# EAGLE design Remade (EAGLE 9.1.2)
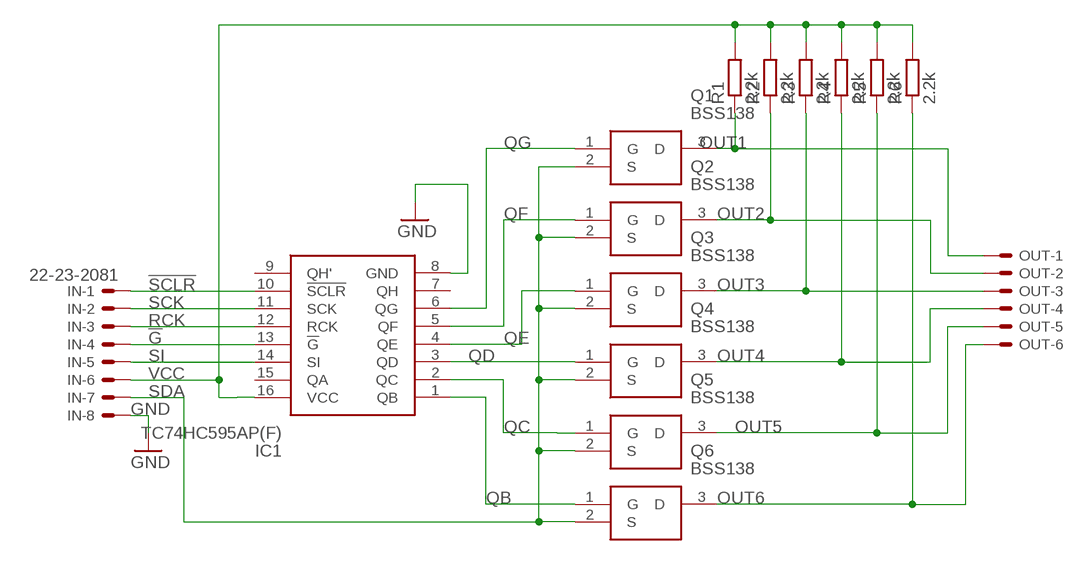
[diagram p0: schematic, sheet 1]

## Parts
IC1  TC74HC595AP(F)  [DIP762W60P254L1925H445Q16N]
IN  22-23-2081  [22-23-2081]
OUT  22-23-2061  [22-23-2061]
Q1  BSS138  [SOT95P240X120-3N]
Q2  BSS138  [SOT95P240X120-3N]
Q3  BSS138  [SOT95P240X120-3N]
Q4  BSS138  [SOT95P240X120-3N]
Q5  BSS138  [SOT95P240X120-3N]
Q6  BSS138  [SOT95P240X120-3N]
R1  2.2k  R-EU_0207/15  [0207/15]
R2  2.2k  R-EU_0207/15  [0207/15]
R3  2.2k  R-EU_0207/15  [0207/15]
R4  2.2k  R-EU_0207/15  [0207/15]
R5  2.2k  R-EU_0207/15  [0207/15]
R6  2.2k  R-EU_0207/15  [0207/15]

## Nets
!G: IC1.13(!G) IN.4
!SCLR: IC1.10(!SCLR) IN.1
GND: IC1.8(GND) IN.8
OUT1: OUT.1 Q1.3(D) R1.1
OUT2: OUT.2 Q2.3(D) R2.1
OUT3: OUT.3 Q3.3(D) R3.1
OUT4: OUT.4 Q4.3(D) R4.1
OUT5: OUT.5 Q5.3(D) R5.1
OUT6: OUT.6 Q6.3(D) R6.1
QB: IC1.1(QB) Q6.1(G)
QC: IC1.2(QC) Q5.1(G)
QD: IC1.3(QD) Q4.1(G)
QE: IC1.4(QE) Q3.1(G)
QF: IC1.5(QF) Q2.1(G)
QG: IC1.6(QG) Q1.1(G)
RCK: IC1.12(RCK) IN.3
SCK: IC1.11(SCK) IN.2
SDA: IN.7 Q1.2(S) Q2.2(S) Q3.2(S) Q4.2(S) Q5.2(S) Q6.2(S)
SI: IC1.14(SI) IN.5
VCC: IC1.16(VCC) IN.6 R1.2 R2.2 R3.2 R4.2 R5.2 R6.2
Unconnected: IC1.7(QH) IC1.9(QH') IC1.15(QA)

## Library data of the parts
IC1 = TC74HC595AP(F):TC74HC595AP(F): IC,CMOS logic,DIP16,SHIFT REGISTERS Source: Datasheet; DESCRIPTION: IC,CMOS logic,DIP16,SHIFT REGISTERS; HEIGHT: 4.45mm; MANUFACTURER_NAME: Toshiba; MANUFACTURER_PART_NUMBER: TC74HC595AP(F); MOUSER_PART_NUMBER: N/A; MOUSER_PRICE-STOCK: https://www.mouser.com/Search/Refine.aspx?Keyword=N%2FA; RS_PART_NUMBER: 5400095P; RS_PRICE-STOCK: http://au.rs-online.com/web/p/products/5400095P
IN = con-molex:22-23-2081: .100" (2.54mm) Center Header - 8 Pin; MF: MOLEX; MPN: 22-23-2081; OC_FARNELL: 1756826; OC_NEWARK: 01C7592
OUT = con-molex:22-23-2061: .100" (2.54mm) Center Header - 6 Pin; MF: MOLEX; MPN: 22-23-2061; OC_FARNELL: 1462922; OC_NEWARK: 27C1933
Q1-Q6 = BSS138:BSS138: N-channel MOSFET,BSS138 0.2A 50V Source: Datasheet; DESCRIPTION: N-channel MOSFET,BSS138 0.2A 50V; HEIGHT: 1.2mm; MANUFACTURER_NAME: ON Semiconductor; MANUFACTURER_PART_NUMBER: BSS138; MOUSER_PART_NUMBER: 512-BSS138; RS_PART_NUMBER: 1241694; RS_PRICE-STOCK: http://uk.rs-online.com/web/p/products/1241694
R1-R6 = rcl:R-EU_: RESISTOR, European symbol; SPICEPREFIX: R

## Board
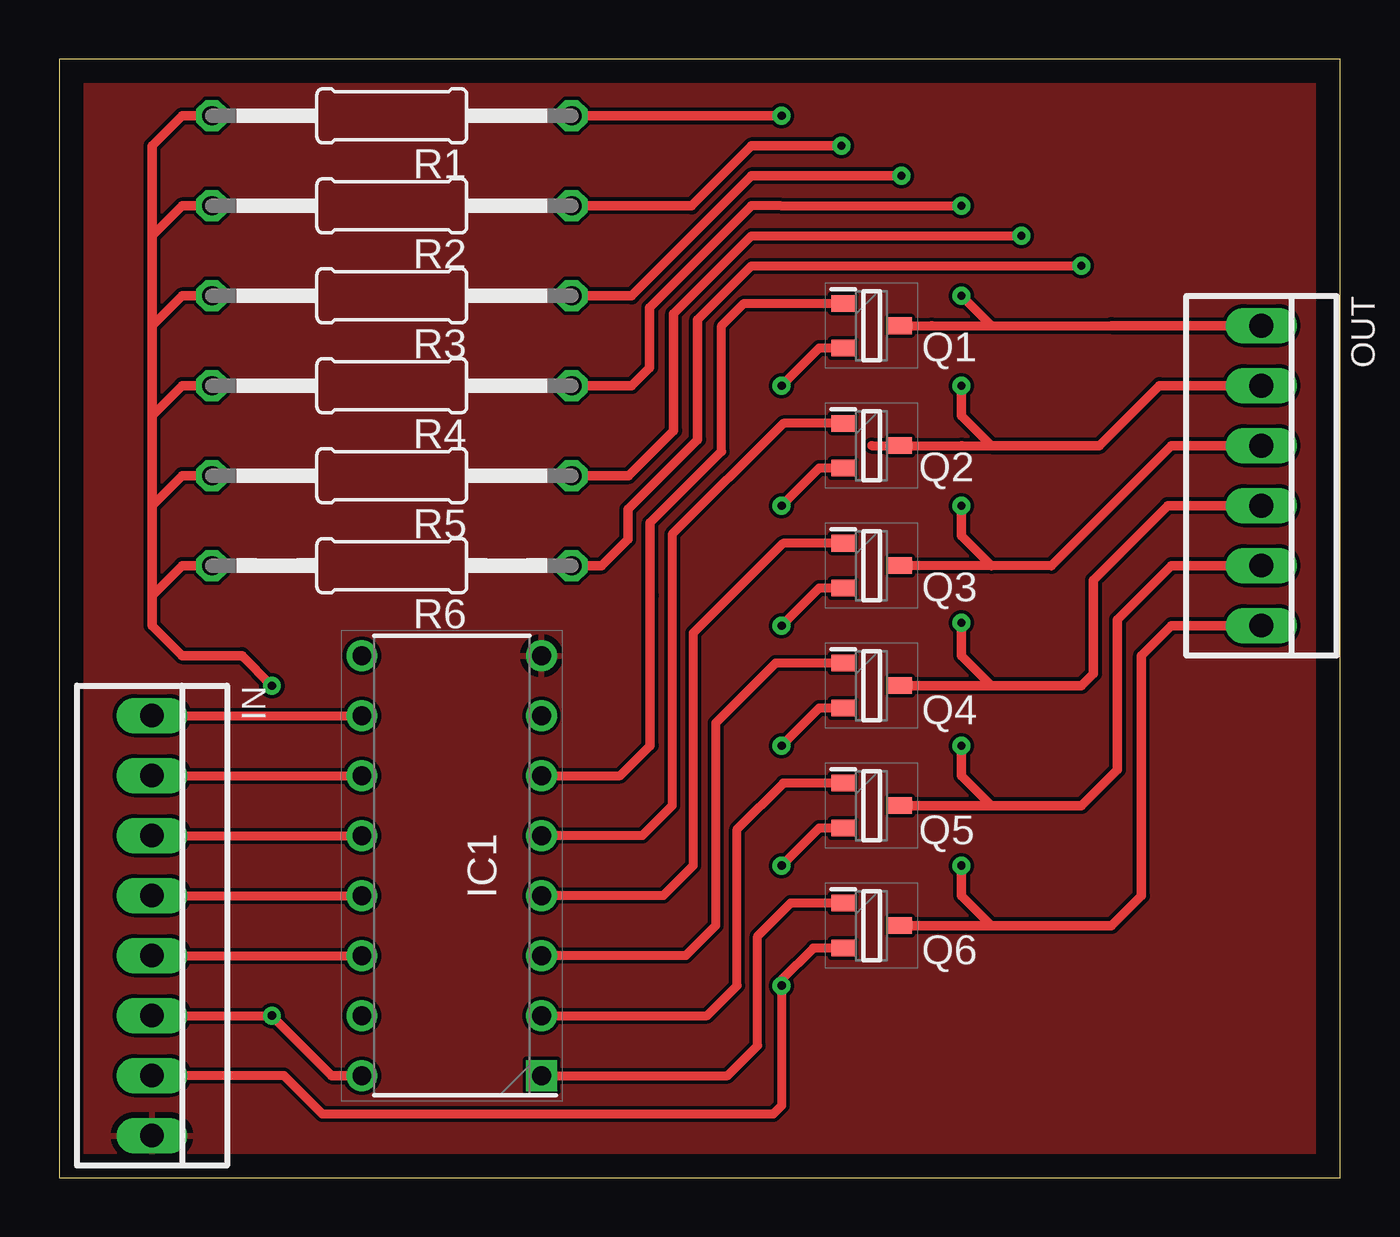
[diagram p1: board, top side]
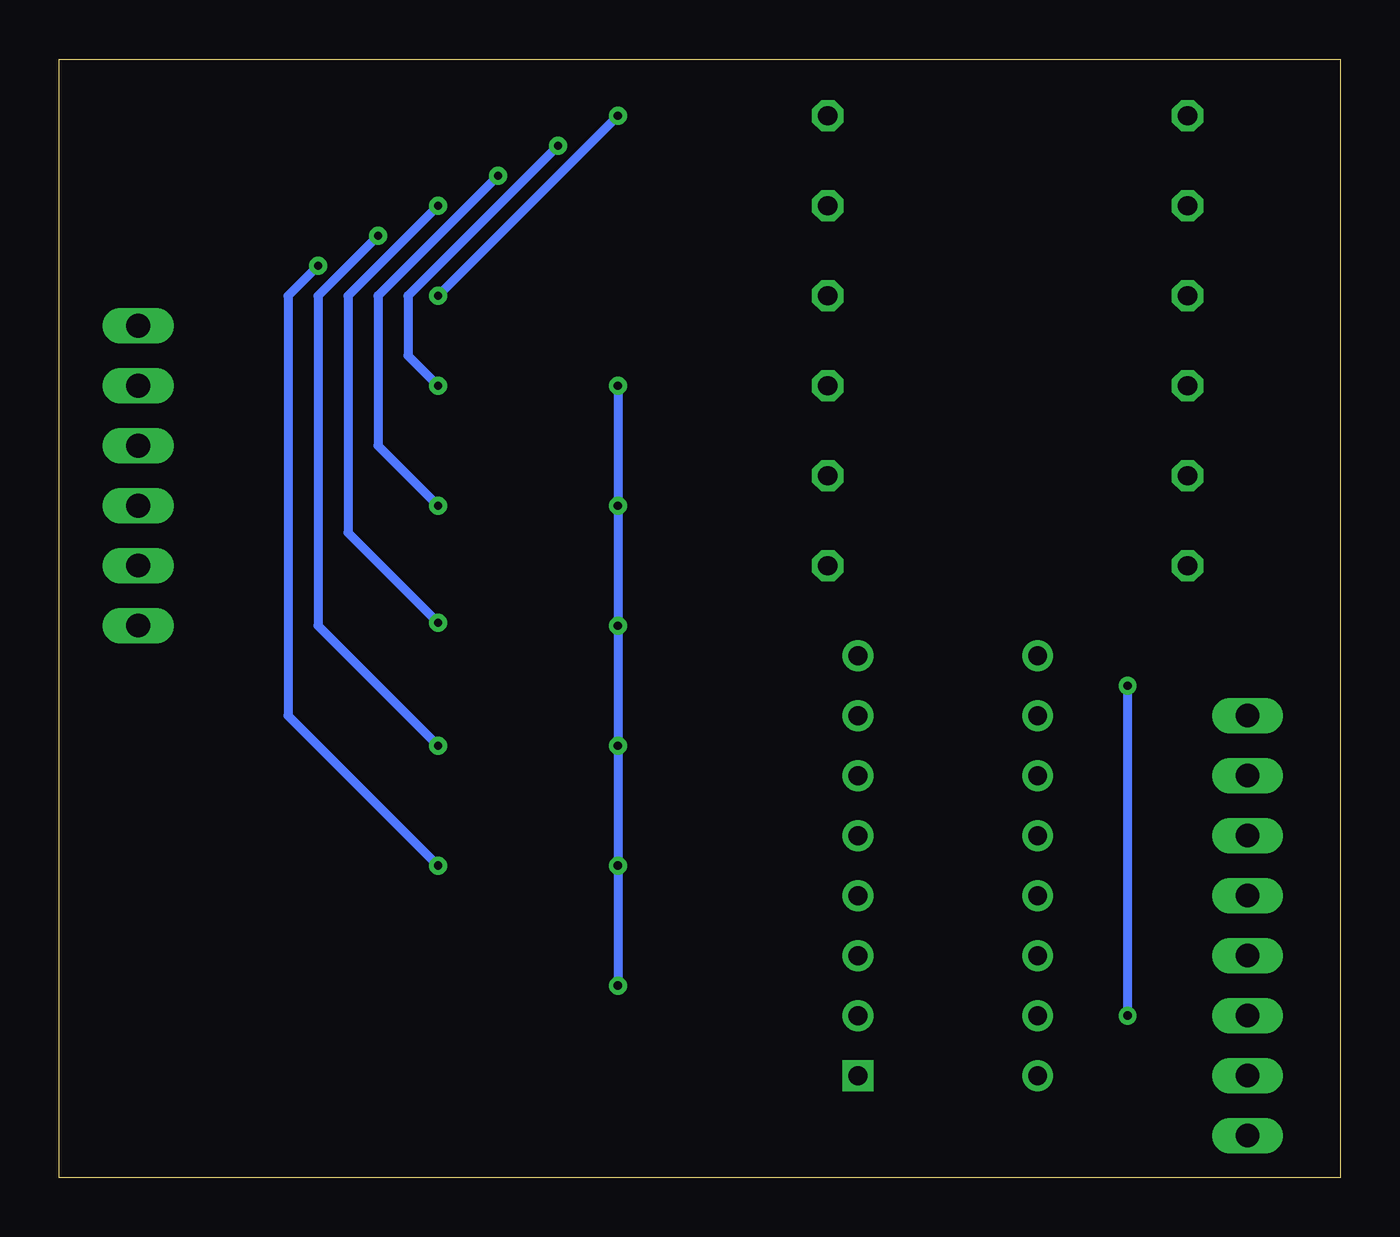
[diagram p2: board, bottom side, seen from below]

Size 54.28 x 47.36 mm. Coordinates in mm from the lower left corner, seen from the top.
Outline: 0,0 54.28,0 54.28,47.36 0,47.36 0,0
Copper layers (1*16): Top 0.035mm / dielectric 1.5mm / Bottom 0.035mm
Design rules "default": minimum track width 6mil, minimum drill 0.35mm, track to track 6mil, track to pad 6mil, pad to pad 6mil, via to via 6mil, smd to smd 6mil, copper to edge 40mil, drill to drill 6mil, minimum pad ring 10mil, minimum via ring 8mil, stop-mask expansion 4mil, vias tented up to drill 0mil, thermal gap 10mil

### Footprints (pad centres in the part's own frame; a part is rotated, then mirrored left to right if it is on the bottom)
DIP762W60P254L1925H445Q16N = drill 0.8 pad 1.2 square: 1 -3.81,8.89 | drill 0.8 pad 1.2: 2 -3.81,6.35; 3 -3.81,3.81; 4 -3.81,1.27; 5 -3.81,-1.27; 6 -3.81,-3.81; 7 -3.81,-6.35; 8 -3.81,-8.89; 9 3.81,-8.89; 10 3.81,-6.35; 11 3.81,-3.81; 12 3.81,-1.27; 13 3.81,1.27; 14 3.81,3.81; 15 3.81,6.35; 16 3.81,8.89
22-23-2081 = drill 1 long: 1 -8.89,0; 2 -6.35,0; 3 -3.81,0; 4 -1.27,0; 5 1.27,0; 6 3.81,0; 7 6.35,0; 8 8.89,0
22-23-2061 = drill 1 long: 1 -6.35,0; 2 -3.81,0; 3 -1.27,0; 4 1.27,0; 5 3.81,0; 6 6.35,0
SOT95P240X120-3N = smd 1 x 0.7: 1 -1.2,0.95; 2 -1.2,-0.95; 3 1.2,0
0207/15 = drill 0.813 octagon: 1 -7.62,0; 2 7.62,0

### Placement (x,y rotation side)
IC1  16.64,13.21 180 top
IN  3.94,10.67 270 top
OUT  50.93,29.72 270 top
Q1  34.42,36.07 0 top
Q2  34.42,30.99 0 top
Q3  34.42,25.91 0 top
Q4  34.42,20.83 0 top
Q5  34.42,15.75 0 top
Q6  34.42,10.67 0 top
R1  14.1,44.96 180 top
R2  14.1,41.15 180 top
R3  14.1,37.34 180 top
R4  14.1,33.53 180 top
R5  14.1,29.72 180 top
R6  14.1,25.91 180 top

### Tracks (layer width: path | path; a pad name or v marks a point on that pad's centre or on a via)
!G
  Top 0.381: IN.4 IC1.13
!SCLR
  Top 0.381: IN.1 IC1.10
GND
  pour Top: -2.41,48.77 -2.41,-0.76 0.13,-3.3 57.28,-3.3 59.82,-0.76 61.09,0.51 61.09,48.77
OUT1  (via drill 0.35)
  Top 0.381: Q1.3 36.96,36.07 39.5,36.07 | 39.5,36.07 44.58,36.07 | v38.23,37.34 39.5,36.07
  Top 0.406: 44.58,36.07 OUT.1 | R1.1 v30.61,44.96
  Bottom 0.381: v30.61,44.96 v38.23,37.34
OUT2  (via drill 0.35)
  Top 0.381: Q2.3 38.23,30.99 | 38.23,30.99 39.5,30.99 | 34.42,30.99 38.23,30.99
  Top 0.406: OUT.2 46.61,33.53 44.07,30.99 39.5,30.99 38.23,32.26 v38.23,33.53 | v33.15,43.69 29.34,43.69 26.8,41.15 R2.1
  Bottom 0.381: 39.5,37.34 39.5,34.8 v38.23,33.53
  Bottom 0.406: v33.15,43.69 39.5,37.34
OUT3  (via drill 0.35)
  Top 0.381: 42.04,25.91 39.5,25.91 Q3.3
  Top 0.406: OUT.3 47.12,30.99 42.04,25.91 | v38.23,28.45 38.23,27.18 39.5,25.91 | v35.69,42.42 29.34,42.42 24.26,37.34 R3.1
  Bottom 0.381: 40.77,37.34 40.77,30.99 v38.23,28.45
  Bottom 0.406: v35.69,42.42 40.77,37.34
OUT4  (via drill 0.35)
  Top 0.381: 35.69,20.83 Q4.3 | 29.34,41.15 30.61,41.15 v38.23,41.15
  Top 0.406: OUT.4 46.96,28.45 43.81,25.3 43.81,21.34 43.31,20.83 39.5,20.83 | 39.5,20.83 35.69,20.83 | v38.23,23.5 38.23,22.1 39.5,20.83 | 29.34,41.15 25.02,36.83 25.02,34.29 24.26,33.53 R4.1
  Bottom 0.381: v38.23,41.15 42.04,37.34 42.04,27.3 v38.23,23.5
OUT5  (via drill 0.35)
  Top 0.381: 26.04,36.58 29.34,39.88 v40.77,39.88
  Top 0.406: OUT.5 47.12,25.91 44.83,23.62 44.83,17.27 43.31,15.75 39.5,15.75 | 39.5,15.75 Q5.3 | v38.23,18.29 38.23,17.02 39.5,15.75 | R5.1 24.13,29.72 26.04,31.62 26.04,36.58
  Bottom 0.381: v38.23,18.29 43.31,23.37 43.31,37.34 v40.77,39.88
OUT6  (via drill 0.35)
  Top 0.381: 35.69,10.67 Q6.3 | 33.47,38.61 34.42,38.61 | 34.42,38.61 v43.31,38.61 | 27.05,36.32 29.34,38.61 34.42,38.61
  Top 0.406: OUT.6 47.12,23.37 45.85,22.1 45.85,11.94 44.58,10.67 43.31,10.67 39.5,10.67 | 39.5,10.67 35.69,10.67 | v38.23,13.21 38.23,11.94 39.5,10.67 | R6.1 22.99,25.91 24.1,27.02 24.1,28.29 27.05,31.24 27.05,36.32
  Bottom 0.381: v43.31,38.61 44.58,37.34 44.58,19.56 v38.23,13.21
QB
  Top 0.381: Q6.1 30.99,11.62 29.59,10.22 29.59,5.59 28.32,4.32 IC1.1
QC
  Top 0.381: Q5.1 30.68,16.7 28.73,14.75 28.73,8.13 27.46,6.86 IC1.2
QD
  Top 0.381: Q4.1 30.35,21.78 27.81,19.24 27.81,10.67 26.54,9.4 IC1.3
QE
  Top 0.381: Q3.1 30.67,26.86 26.86,23.05 26.86,13.21 25.59,11.94 IC1.4
QF
  Top 0.381: Q2.1 30.68,31.94 25.97,27.23 25.97,15.75 24.7,14.48 IC1.5
QG
  Top 0.381: 25.04,18.29 23.77,17.02 IC1.6 | 25.04,27.72 28.07,30.74 28.07,36.07 29.02,37.02 Q1.1
  Top 0.406: 25.04,18.29 25.04,24.64 25.04,27.72
RCK
  Top 0.381: IN.3 IC1.12
SCK
  Top 0.381: IN.2 IC1.11
SDA  (via drill 0.35)
  Top 0.381: IN.7 9.53,4.32 11.17,2.69 30.24,2.69 30.61,3.05 v30.61,8.13 30.61,8.38 31.95,9.72 Q6.2 | Q2.2 32.2,30.04 v30.61,28.45 | Q3.2 32.2,24.96 v30.61,23.37 | Q4.2 32.2,19.88 v30.61,18.29 | Q5.2 32.2,14.8 v30.61,13.21 | Q1.2 32.2,35.12 v30.61,33.53
  Bottom 0.381: v30.61,33.53 v30.61,28.45 v30.61,23.37 v30.61,18.29 v30.61,13.21 v30.61,8.13
SI
  Top 0.381: IN.5 IC1.14
VCC  (via drill 0.35)
  Top 0.381: IN.6 v9.02,6.86
  Top 0.406: v9.02,6.86 11.56,4.32 IC1.16 | v9.02,20.83 7.75,22.1 5.21,22.1 3.94,23.37 3.94,24.64 | 3.94,24.64 3.94,28.45 | 3.94,28.45 3.94,32.26 | 3.94,32.26 3.94,36.07 | 3.94,36.07 3.94,39.88 | 3.94,39.88 3.94,43.69 5.21,44.96 R1.2 | 3.94,39.88 5.21,41.15 R2.2 | 3.94,36.07 5.21,37.34 R3.2 | 3.94,32.26 5.21,33.53 R4.2 | 3.94,28.45 5.21,29.72 R5.2 | 3.94,24.64 5.21,25.91 R6.2
  Bottom 0.381: v9.02,6.86 v9.02,20.83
